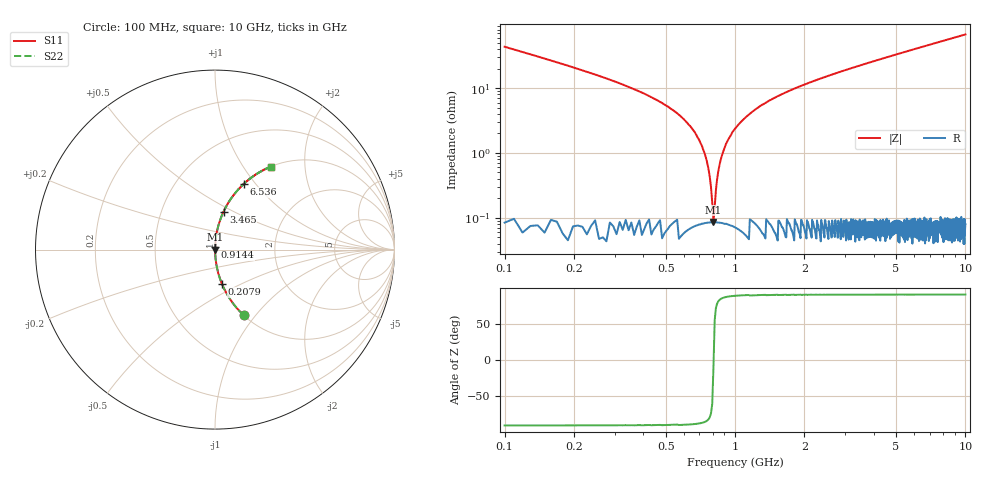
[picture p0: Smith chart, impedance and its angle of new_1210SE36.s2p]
!	AVX	Thin	Film	Operation	Date:	April 2007
!	Description:	Accu-P®	"Series,"	Thin	"Film,"	"SMD,"	RF	Capacitor
!	Part	Number:	12101J360FBT
!	100	MHz	-	5.05	GHz
!	Serial	Measurements
#	MHZ	S	MA	R	50
!	S11	S21	S12	S22
!	dB	Phase	dB	Phase	dB	Phase	dB	Phase
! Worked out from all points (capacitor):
!   1010 points, 100 MHz to 10 GHz, reference 50 ohm
!   read as one part in series: C = 36 pF near 149.1 MHz
!   lowest |Z| = 86.1 mohm at 806.4 MHz (marker M1)
!   series resonance near 807.4 MHz, so ESL is about 1.1 nH
!   S11 on the Smith chart (normalised r, x): 100 MHz: 1.00, -0.87; 207.9 MHz: 1.00, -0.40; 914.4 MHz: 1.00, +0.03; 3.465 GHz: 1.00, +0.44; 6.536 GHz: 1.00, +0.87; 10 GHz: 1.00, +1.35
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100  0.399 -66.4  0.916 23.5  0.916 23.5  0.399 -66.4
207.929  0.195 -78.6  0.98 11.2  0.98 11.2  0.195 -78.6
629.832  0.027 -87.0  0.999 1.6  0.999 1.6  0.027 -87.0
708.325  0.014 -86.4  0.999 0.8  0.999 0.8  0.014 -86.4
737.76  0.00991 -85.4  0.999 0.6  0.999 0.6  0.00991 -85.4
767.195  0.00564 -82.6  0.999 0.3  0.999 0.3  0.00564 -82.6
806.442  0.000713 -11.0  0.999 0.0  0.999 0.0  0.000713 -11.0
845.689  0.00511 81.8  0.999 -0.3  0.999 -0.3  0.00511 81.8
875.124  0.00885 85.0  0.999 -0.5  0.999 -0.5  0.00885 85.0
914.371  0.014 86.3  0.999 -0.8  0.999 -0.8  0.014 86.3
1022.299  0.026 87.0  0.999 -1.5  0.999 -1.5  0.026 87.0
1198.91  0.044 86.6  0.998 -2.5  0.998 -2.5  0.044 86.6
1434.39  0.066 85.6  0.997 -3.8  0.997 -3.8  0.066 85.6
1758.176  0.094 84.2  0.995 -5.4  0.995 -5.4  0.094 84.2
2474.43  0.148 81.2  0.988 -8.5  0.988 -8.5  0.148 81.2
3406.541  0.213 77.5  0.976 -12.3  0.976 -12.3  0.213 77.5
3465.411  0.217 77.3  0.976 -12.5  0.976 -12.5  0.217 77.3
5054.906  0.317 71.4  0.948 -18.5  0.948 -18.5  0.317 71.4
6536.472  0.4 66.3  0.916 -23.6  0.916 -23.6  0.4 66.3
6703.271  0.409 65.8  0.912 -24.1  0.912 -24.1  0.409 65.8
8351.635  0.489 60.7  0.872 -29.3  0.872 -29.3  0.489 60.7
10000  0.558 56.0  0.829 -33.9  0.829 -33.9  0.558 56.0
